| TEXAS INSTRUMENTS INCORPORATED
| Standard Linear and Logic Group
| IBIS Model of SN74LVT8986
| 3.3-V LINKING ADDRESSABLE SCAN PORTS
| MULTIDROP-ADDRESSABLE IEEE STD 1149.1 (JTAG) TAP TRANSCEIVERS
| This file contains package information for the following:
|  PBGS 64-pin (GGV) package as [Component] LVT8986_GGV
|  LQFP 64-pin (PM) package as [Component] LVT8986_PM
|  CFP 64-pin (HV) package as [Component] LVT8986_HV
| This device can be powered at the following Vccs:
|  3.3 volt Vcc
| This file provides unique models under the [Model Selector] for each Vcc.
| For operation at a specific Vcc, select the appropriate model after each
| [Model Selector] keyword.
[IBIS Ver]   3.2
[Comment char]  |_char
[File Name]   sn74lvt8986.ibs
[File Rev]   1.0 | a_die
[Date]   September 4, 2008
[Source]   Data created from TI-SPICE simulations at TI-SLL.
[Notes]   The following is an IBIS list for the LVT8986.
   Please contact sllibis@ti.com with questions and
   comments concerning SLL IBIS models.
   NOTE:  The gnd_clamp, pwr_clamp, pullup, and pulldown data
   for ranges beyond GND-VCC may have modeling inaccuracies due
   to convergence problems over the extended IBIS ranges.
|   FILE REV HISTORY
[Disclaimer] Property of Texas Instruments Incorporated.  Unauthorized
   reproduction and/or distribution is strictly prohibited.
   This product is protected under copyright law.
   Created  2002, (C) Copyright  2002, Texas Instruments
   Incorporated, All Rights Reserved
   UNLESS THERE IS A SIGNED, WRITTEN AGREEMENT TO THE
   CONTRARY, TEXAS INSTRUMENTS (TI) IS PROVIDING THE IBIS
   MODELS  AND WITHOUT ANY WARRANTY, EXPRESSED OR
   IMPLIED.  TI assumes no liability for:
   1) the accuracy of the IBIS models provided to your
   company;
   2) the proper functioning of these IBIS Models in your
   design or for any resulting applications; or
   3) infringement of patents, copyrights or intellectual
   property rights resulting from your use of these IBIS
   models.
   TI provides IBIS Models as a service to our customers.
   You and your company shall not distribute, sell or give
   these models to anyone else without prior written
   permission from TI.
   TI reserves the right to make changes to our products or
   to discontinue any semiconductor product or service
   without notice, and advises our customers to obtain the
   latest version of relevant information to verify, before
   placing orders, that the information being relied on is
   current.
   Please be aware that your receipt and use of the IBIS
   information provided shall serve as acceptance of these
   terms and conditions.  If you do not accept these terms,
   you should return or destroy the IBIS models and any
   other accompanying information immediately.
| Component LVT8986_GGV 64-pin PBGA
[Component]   LVT8986_GGV
[Manufacturer]   Texas Instruments, Inc.
[Package]
|   typ   min   max
R_pkg   7.900e-02   6.900e-02   1.010e-01
L_pkg   3.757e-09   1.665e-09   4.658e-09
C_pkg   5.510e-13   1.220e-13   6.540e-13
[Pin]   signal_name   model_name   R_pin   L_pin   C_pin
1A   A0   LVT8986_PU_IN   8.500e-02   4.537e-09   5.660e-13
1B   A1   LVT8986_PU_IN   8.500e-02   4.357e-09   6.400e-13
1C   GND   GND   8.500e-02   4.094e-09   6.210e-13
1D   A5   LVT8986_PU_IN   8.400e-02   3.770e-09   5.570e-13
1E   A8   LVT8986_PU_IN   8.500e-02   3.778e-09   5.600e-13
1F   P0   LVT8986_PU_IN   8.500e-02   3.935e-09   5.840e-13
1G   VCC   POWER   7.100e-02   3.797e-09   5.980e-13
1H   NBYP1   LVT8986_PU_IN   8.700e-02   4.341e-09   5.690e-13
2A   NSTRST0   LVT8986_OUT   7.100e-02   3.838e-09   5.990e-13
2B   NOE   LVT8986_PTCK_IN   8.900e-02   4.400e-09   5.770e-13
2C   A2   LVT8986_PU_IN   8.500e-02   4.193e-09   6.290e-13
2D   A6   LVT8986_PU_IN   8.500e-02   3.744e-09   5.260e-13
2E   A7   LVT8986_PU_IN   8.500e-02   3.738e-09   5.470e-13
2F   P1   LVT8986_PU_IN   8.500e-02   4.080e-09   6.200e-13
2G   NBYP0   LVT8986_PU_IN   8.500e-02   4.492e-09   5.850e-13
2H   NBYP2   LVT8986_PU_IN   7.000e-02   3.792e-09   5.980e-13
3A   GND   GND   7.100e-02   3.597e-09   5.760e-13
3B   STMS0   LVT8986_OUT   7.100e-02   3.600e-09   5.800e-13
3C   STCK0   LVT8986_OUT   7.100e-02   3.678e-09   5.890e-13
3D   A4   LVT8986_PU_IN   8.500e-02   3.858e-09   5.710e-13
3E   A9   LVT8986_PU_IN   8.500e-02   3.837e-09   5.700e-13
3F   P2   LVT8986_PU_IN   8.600e-02   4.193e-09   6.280e-13
3G   NBYP3   LVT8986_PU_IN   7.100e-02   3.671e-09   5.910e-13
3H   NBYP4   LVT8986_PU_IN   7.100e-02   3.581e-09   5.840e-13
4A   STDO0   LVT8986_TRI   7.100e-02   3.412e-09   5.260e-13
4B   SY0   LVT8986_OUT   7.200e-02   3.487e-09   5.320e-13
4C   STDI0   LVT8986_PU_IN   7.100e-02   3.449e-09   5.350e-13
4D   A3   LVT8986_PU_IN   8.500e-02   3.956e-09   5.850e-13
4E   NBYP5   LVT8986_PU_IN   7.000e-02   3.480e-09   5.430e-13
4F   NPTRST   LVT8986_PU2_IN   7.000e-02   3.469e-09   5.330e-13
4G   PTMS   LVT8986_PU2_IN   7.100e-02   3.408e-09   5.020e-13
4H   PTCK   LVT8986_PTCK_IN   7.100e-02   3.424e-09   5.330e-13
5A   SX0   LVT8986_PU_IN   7.100e-02   3.413e-09   5.220e-13
5B   VCC   POWER   8.500e-02   4.302e-09   6.360e-13
5C   NCON0   LVT8986_OUT   7.100e-02   3.452e-09   5.310e-13
5D   NSTRST1   LVT8986_OUT   7.100e-02   3.482e-09   5.430e-13
5E   GND   GND   8.500e-02   3.942e-09   5.840e-13
5F   PTDO   LVT8986_TRI   7.200e-02   3.551e-09   5.460e-13
5G   PTDI   LVT8986_PU2_IN   7.000e-02   3.428e-09   5.170e-13
5H   CTDI   LVT8986_PU2_IN   7.000e-02   3.439e-09   5.350e-13
6A   GND   GND   8.500e-02   3.971e-09   5.890e-13
6B   STCK1   LVT8986_OUT   7.100e-02   3.636e-09   5.850e-13
6C   SY1   LVT8986_OUT   8.500e-02   4.260e-09   6.400e-13
6D   NCON1   LVT8986_OUT   8.600e-02   3.886e-09   5.750e-13
6E   STDI2   LVT8986_PU_IN   8.500e-02   3.843e-09   5.690e-13
6F   PY   LVT8986_OUT   7.100e-02   3.685e-09   5.930e-13
6G   GND   GND   7.200e-02   3.566e-09   5.800e-13
6H   CTDO   LVT8986_TRI   7.000e-02   3.630e-09   5.540e-13
7A   STMS1   LVT8986_OUT   8.400e-02   4.025e-09   6.070e-13
7B   VCC   POWER   7.200e-02   3.488e-09   5.060e-13
7C   GND   GND   7.000e-02   3.505e-09   5.440e-13
7D   VCC   POWER   8.500e-02   4.632e-09   6.080e-13
7E   STCK2   LVT8986_OUT   8.600e-02   3.832e-09   5.380e-13
7F   SY2   LVT8986_OUT   8.600e-02   4.189e-09   6.290e-13
7G   PX   LVT8986_PU_IN   8.900e-02   4.378e-09   5.730e-13
7H   VCC   POWER   8.500e-02   3.837e-09   5.600e-13
8A   STDI1   LVT8986_PU_IN   1.010e-01   4.658e-09   5.900e-13
8B   STDO1   LVT8986_TRI   8.500e-02   4.413e-09   6.540e-13
8C   SX1   LVT8986_PU_IN   8.500e-02   4.131e-09   6.260e-13
8D   NSTRST2   LVT8986_OUT   8.600e-02   3.846e-09   5.730e-13
8E   STMS2   LVT8986_OUT   8.500e-02   3.824e-09   5.690e-13
8F   STDO2   LVT8986_TRI   8.600e-02   4.084e-09   6.210e-13
8G   SX2   LVT8986_PU_IN   8.500e-02   4.310e-09   6.360e-13
8H   NCON2   LVT8986_OUT   8.500e-02   4.496e-09   5.880e-13
| Component LVT8986_PM 64-pin LQFP
[Component]   LVT8986_PM
[Manufacturer]   Texas Instruments, Inc.
[Package]
|   typ   min   max
R_pkg   7.900e-02   6.900e-02   1.010e-01
L_pkg   3.757e-09   1.665e-09   4.658e-09
C_pkg   5.510e-13   1.220e-13   6.540e-13
[Pin]   signal_name   model_name   R_pin   L_pin   C_pin
1   A0   LVT8986_PU_IN   8.500e-02   4.537e-09   5.660e-13
2   A1   LVT8986_PU_IN   8.500e-02   4.357e-09   6.400e-13
3   A2   LVT8986_PU_IN   8.500e-02   4.193e-09   6.290e-13
4   GND   GND   8.500e-02   4.094e-09   6.210e-13
5   A3   LVT8986_PU_IN   8.500e-02   3.956e-09   5.850e-13
6   A4   LVT8986_PU_IN   8.500e-02   3.858e-09   5.710e-13
7   A5   LVT8986_PU_IN   8.400e-02   3.770e-09   5.570e-13
8   A6   LVT8986_PU_IN   8.500e-02   3.744e-09   5.260e-13
9   A7   LVT8986_PU_IN   8.500e-02   3.738e-09   5.470e-13
10   A8   LVT8986_PU_IN   8.500e-02   3.778e-09   5.600e-13
11   A9   LVT8986_PU_IN   8.500e-02   3.837e-09   5.700e-13
12   P0   LVT8986_PU_IN   8.500e-02   3.935e-09   5.840e-13
13   P1   LVT8986_PU_IN   8.500e-02   4.080e-09   6.200e-13
14   P2   LVT8986_PU_IN   8.600e-02   4.193e-09   6.280e-13
15   VCC   POWER   8.500e-02   4.302e-09   6.360e-13
16   NBYP0   LVT8986_PU_IN   8.500e-02   4.492e-09   5.850e-13
17   NBYP1   LVT8986_PU_IN   8.700e-02   4.341e-09   5.690e-13
18   NBYP2   LVT8986_PU_IN   7.000e-02   3.792e-09   5.980e-13
19   NBYP3   LVT8986_PU_IN   7.100e-02   3.671e-09   5.910e-13
20   NBYP4   LVT8986_PU_IN   7.100e-02   3.581e-09   5.840e-13
21   NBYP5   LVT8986_PU_IN   7.000e-02   3.480e-09   5.430e-13
22   NPTRST   LVT8986_PU2_IN   7.000e-02   3.469e-09   5.330e-13
23   PTCK   LVT8986_PTCK_IN   7.100e-02   3.424e-09   5.330e-13
24   PTMS   LVT8986_PU2_IN   7.100e-02   3.408e-09   5.020e-13
25   PTDI   LVT8986_PU2_IN   7.000e-02   3.428e-09   5.170e-13
26   CTDI   LVT8986_PU2_IN   7.000e-02   3.439e-09   5.350e-13
27   PTDO   LVT8986_TRI   7.200e-02   3.551e-09   5.460e-13
28   CTDO   LVT8986_TRI   7.000e-02   3.630e-09   5.540e-13
29   GND   GND   7.100e-02   3.597e-09   5.760e-13
30   PY   LVT8986_OUT   7.100e-02   3.685e-09   5.930e-13
31   VCC   POWER   7.100e-02   3.797e-09   5.980e-13
32   PX   LVT8986_PU_IN   8.900e-02   4.378e-09   5.730e-13
33   NCON2   LVT8986_OUT   8.500e-02   4.496e-09   5.880e-13
34   SX2   LVT8986_PU_IN   8.500e-02   4.310e-09   6.360e-13
35   SY2   LVT8986_OUT   8.600e-02   4.189e-09   6.290e-13
36   STDO2   LVT8986_TRI   8.600e-02   4.084e-09   6.210e-13
37   GND   GND   8.500e-02   3.942e-09   5.840e-13
38   STDI2   LVT8986_PU_IN   8.500e-02   3.843e-09   5.690e-13
39   STMS2   LVT8986_OUT   8.500e-02   3.824e-09   5.690e-13
40   STCK2   LVT8986_OUT   8.600e-02   3.832e-09   5.380e-13
41   VCC   POWER   8.500e-02   3.837e-09   5.600e-13
42   NSTRST2   LVT8986_OUT   8.600e-02   3.846e-09   5.730e-13
43   NCON1   LVT8986_OUT   8.600e-02   3.886e-09   5.750e-13
44   GND   GND   8.500e-02   3.971e-09   5.890e-13
45   SX1   LVT8986_PU_IN   8.500e-02   4.131e-09   6.260e-13
46   SY1   LVT8986_OUT   8.500e-02   4.260e-09   6.400e-13
47   STDO1   LVT8986_TRI   8.500e-02   4.413e-09   6.540e-13
48   VCC   POWER   8.500e-02   4.632e-09   6.080e-13
49   STDI1   LVT8986_PU_IN   1.010e-01   4.658e-09   5.900e-13
50   STMS1   LVT8986_OUT   8.400e-02   4.025e-09   6.070e-13
51   STCK1   LVT8986_OUT   7.100e-02   3.636e-09   5.850e-13
52   GND   GND   7.200e-02   3.566e-09   5.800e-13
53   NSTRST1   LVT8986_OUT   7.100e-02   3.482e-09   5.430e-13
54   NCON0   LVT8986_OUT   7.100e-02   3.452e-09   5.310e-13
55   SX0   LVT8986_PU_IN   7.100e-02   3.413e-09   5.220e-13
56   VCC   POWER   7.200e-02   3.488e-09   5.060e-13
57   SY0   LVT8986_OUT   7.200e-02   3.487e-09   5.320e-13
58   STDO0   LVT8986_TRI   7.100e-02   3.412e-09   5.260e-13
59   STDI0   LVT8986_PU_IN   7.100e-02   3.449e-09   5.350e-13
60   GND   GND   7.000e-02   3.505e-09   5.440e-13
61   STMS0   LVT8986_OUT   7.100e-02   3.600e-09   5.800e-13
62   STCK0   LVT8986_OUT   7.100e-02   3.678e-09   5.890e-13
63   NSTRST0   LVT8986_OUT   7.100e-02   3.838e-09   5.990e-13
64   NOE   LVT8986_PTCK_IN   8.900e-02   4.400e-09   5.770e-13
| Component LVT8986_HV 64-pin CFP
[Component]   LVT8986_HV
[Manufacturer]   Texas Instruments, Inc.
[Package]
|   typ   min   max
R_pkg   7.900e-02   6.900e-02   1.010e-01
L_pkg   3.757e-09   1.665e-09   4.658e-09
C_pkg   5.510e-13   1.220e-13   6.540e-13
[Pin]   signal_name   model_name   R_pin   L_pin   C_pin
1   NC   NC
2   SY0   LVT8986_OUT   7.200e-02   3.487e-09   5.320e-13
3   STDO0   LVT8986_TRI   7.100e-02   3.412e-09   5.260e-13
4   STDI0   LVT8986_PU_IN   7.100e-02   3.449e-09   5.350e-13
5   GND   GND   7.000e-02   3.505e-09   5.440e-13
6   STMS0   LVT8986_OUT   7.100e-02   3.600e-09   5.800e-13
7   STCK0   LVT8986_OUT   7.100e-02   3.678e-09   5.890e-13
8   NSTRST0   LVT8986_OUT   7.100e-02   3.838e-09   5.990e-13
9   NOE   LVT8986_PTCK_IN   8.900e-02   4.400e-09   5.770e-13
10   A0   LVT8986_PU_IN   8.500e-02   4.537e-09   5.660e-13
11   A1   LVT8986_PU_IN   8.500e-02   4.357e-09   6.400e-13
12   A2   LVT8986_PU_IN   8.500e-02   4.193e-09   6.290e-13
13   GND   GND   8.500e-02   4.094e-09   6.210e-13
14   A3   LVT8986_PU_IN   8.500e-02   3.956e-09   5.850e-13
15   A4   LVT8986_PU_IN   8.500e-02   3.858e-09   5.710e-13
16   A5   LVT8986_PU_IN   8.400e-02   3.770e-09   5.570e-13
17   A6   LVT8986_PU_IN   8.500e-02   3.744e-09   5.260e-13
18   NC   NC
19   A7   LVT8986_PU_IN   8.500e-02   3.738e-09   5.470e-13
20   A8   LVT8986_PU_IN   8.500e-02   3.778e-09   5.600e-13
21   A9   LVT8986_PU_IN   8.500e-02   3.837e-09   5.700e-13
22   P0   LVT8986_PU_IN   8.500e-02   3.935e-09   5.840e-13
23   P1   LVT8986_PU_IN   8.500e-02   4.080e-09   6.200e-13
24   P2   LVT8986_PU_IN   8.600e-02   4.193e-09   6.280e-13
25   VCC   POWER   8.500e-02   4.302e-09   6.360e-13
26   NBYP0   LVT8986_PU_IN   8.500e-02   4.492e-09   5.850e-13
27   NBYP1   LVT8986_PU_IN   8.700e-02   4.341e-09   5.690e-13
28   NBYP2   LVT8986_PU_IN   7.000e-02   3.792e-09   5.980e-13
29   NBYP3   LVT8986_PU_IN   7.100e-02   3.671e-09   5.910e-13
30   NBYP4   LVT8986_PU_IN   7.100e-02   3.581e-09   5.840e-13
31   NBYP5   LVT8986_PU_IN   7.000e-02   3.480e-09   5.430e-13
32   NPTRST   LVT8986_PU2_IN   7.000e-02   3.469e-09   5.330e-13
33   PTCK   LVT8986_PTCK_IN   7.100e-02   3.424e-09   5.330e-13
34   PTMS   LVT8986_PU2_IN   7.100e-02   3.408e-09   5.020e-13
35   NC   NC
36   PTDI   LVT8986_PU2_IN   7.000e-02   3.428e-09   5.170e-13
37   CTDI   LVT8986_PU2_IN   7.000e-02   3.439e-09   5.350e-13
38   PTDO   LVT8986_TRI   7.200e-02   3.551e-09   5.460e-13
39   CTDO   LVT8986_TRI   7.000e-02   3.630e-09   5.540e-13
40   GND   GND   7.100e-02   3.597e-09   5.760e-13
41   PY   LVT8986_OUT   7.100e-02   3.685e-09   5.930e-13
42   VCC   POWER   7.100e-02   3.797e-09   5.980e-13
43   PX   LVT8986_PU_IN   8.900e-02   4.378e-09   5.730e-13
44   NCON2   LVT8986_OUT   8.500e-02   4.496e-09   5.880e-13
45   SX2   LVT8986_PU_IN   8.500e-02   4.310e-09   6.360e-13
46   SY2   LVT8986_OUT   8.600e-02   4.189e-09   6.290e-13
47   STDO2   LVT8986_TRI   8.600e-02   4.084e-09   6.210e-13
48   GND   GND   8.500e-02   3.942e-09   5.840e-13
49   STDI2   LVT8986_PU_IN   8.500e-02   3.843e-09   5.690e-13
50   STMS2   LVT8986_OUT   8.500e-02   3.824e-09   5.690e-13
51   STCK2   LVT8986_OUT   8.600e-02   3.832e-09   5.380e-13
52   NC   NC
53   VCC   POWER   8.500e-02   3.837e-09   5.600e-13
54   NSTRST2   LVT8986_OUT   8.600e-02   3.846e-09   5.730e-13
55   NCON1   LVT8986_OUT   8.600e-02   3.886e-09   5.750e-13
56   GND   GND   8.500e-02   3.971e-09   5.890e-13
57   SX1   LVT8986_PU_IN   8.500e-02   4.131e-09   6.260e-13
58   SY1   LVT8986_OUT   8.500e-02   4.260e-09   6.400e-13
59   STDO1   LVT8986_TRI   8.500e-02   4.413e-09   6.540e-13
60   VCC   POWER   8.500e-02   4.632e-09   6.080e-13
61   STDI1   LVT8986_PU_IN   1.010e-01   4.658e-09   5.900e-13
62   STMS1   LVT8986_OUT   8.400e-02   4.025e-09   6.070e-13
63   STCK1   LVT8986_OUT   7.100e-02   3.636e-09   5.850e-13
64   GND   GND   7.200e-02   3.566e-09   5.800e-13
65   NSTRST1   LVT8986_OUT   7.100e-02   3.482e-09   5.430e-13
66   NCON0   LVT8986_OUT   7.100e-02   3.452e-09   5.310e-13
67   SX0   LVT8986_PU_IN   7.100e-02   3.413e-09   5.220e-13
68   VCC   POWER   7.200e-02   3.488e-09   5.060e-13
| Model LVT8986_PU2_IN
[Model Selector]   LVT8986_PU2_IN
LVT8986_PU2_IN_33B   3.3 volt Vcc
| Model LVT8986_PTCK_IN
[Model Selector]   LVT8986_PTCK_IN
LVT8986_PTCK_IN_33B   3.3 volt Vcc
| Model LVT8986_PU_IN
[Model Selector]   LVT8986_PU_IN
LVT8986_PU_IN_33B   3.3 volt Vcc
| Model LVT8986_OUT
[Model Selector]   LVT8986_OUT
LVT8986_OUT_33B   3.3 volt Vcc
| Model LVT8986_TRI
[Model Selector]   LVT8986_TRI
LVT8986_TRI_33B   3.3 volt Vcc
| Models and submodels in the file (5): LVT8986_PU2_IN_33B (Input), LVT8986_PTCK_IN_33B (Input), LVT8986_PU_IN_33B (Input), LVT8986_OUT_33B (Output), LVT8986_TRI_33B (3-state)
